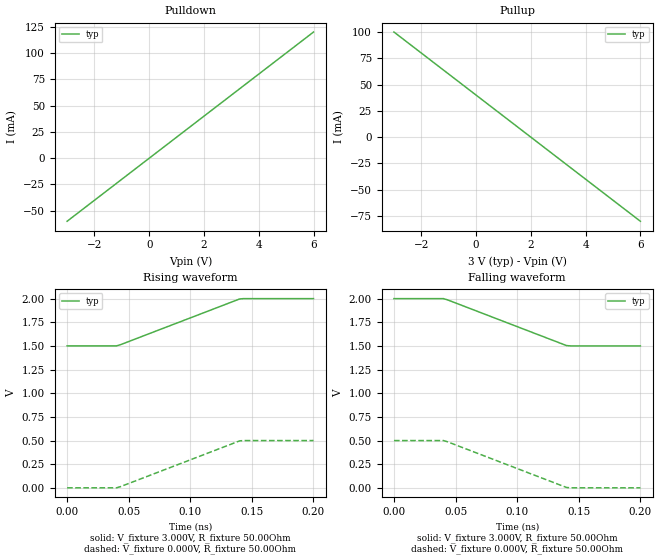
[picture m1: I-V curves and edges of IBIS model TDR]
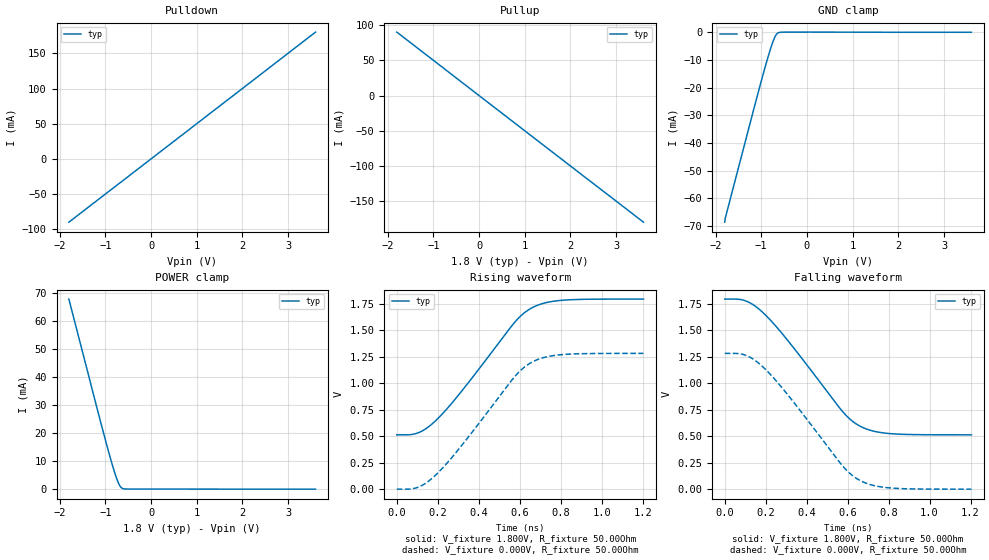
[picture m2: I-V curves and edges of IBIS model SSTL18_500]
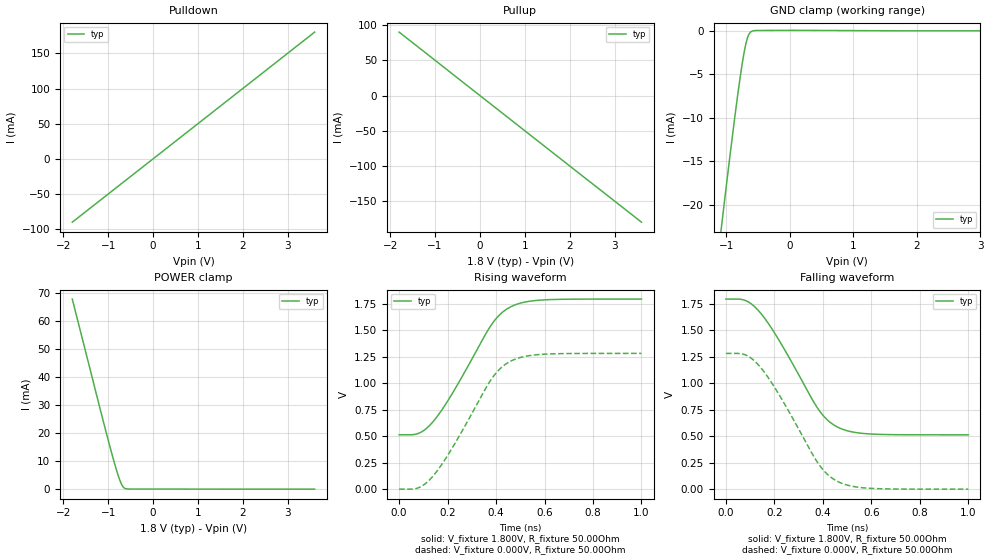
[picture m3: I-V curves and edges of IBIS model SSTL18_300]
[IBIS Ver]   3.2
[File Name]   bogatin_lab.ibs
[File Rev]   0.00
[Date]   10/29/2003
[Source]   Arpad Muranyi, Mentor Graphics
[Notes]   These models were made from the HyperLynx .MOD libraries
[Disclaimer]   This information is for educational purposes only.
[Copyright]   Copyright 2013, Mentor Graphics.  All Rights Reserved.
[Component]   Bogatin_Lab
[Manufacturer]  Mentor Graphics Corporation
[Package]
|   typ   min   max
R_pkg   0.00Ohm   0.00Ohm   0.00Ohm
L_pkg   0.00nH   0.00nH   0.00nH
C_pkg   0.00pF   0.00pF   0.00pF
[PIN]   signal_name   model_name   R_pin   L_pin   C_pin
1   Vcc   Power
2   GND   GND
3   TDR   TDR   10.000mOhm   2.000nH   0.800pF
4   SSTL18_500   SSTL18_500   10.000mOhm   0.050nH   0.050pF
5   SSTL18_300   SSTL18_300   10.000mOhm   0.050nH   0.050pF
6   SSTL18_200   SSTL18_200   10.000mOhm   0.050nH   0.050pF
7   CMOS33_UF8   CMOS33_UF8   10.000mOhm   0.050nH   0.050pF
8   CMOS33_UF_P   CMOS33_UF8   10.000mOhm   0.050nH   0.050pF
9   CMOS33_UF_N   CMOS33_UF8   10.000mOhm   0.050nH   0.050pF
10   CMOS33_UF4   CMOS33_UF4   10.000mOhm   2.000nH   0.800pF
11   CMOS33_UF4   CMOS33_UF4   10.000mOhm   0.050nH   0.050pF
12   CMOS33_MED8   CMOS33_MED8   10.000mOhm   0.050nH   0.050pF
13   CMOS33_MED4   CMOS33_MED4   10.000mOhm   0.050nH   0.050pF
14   SSTL25_01ns   SSTL25_01ns   10.000mOhm   0.050nH   0.050pF
[Diff Pin]  inv_pin  vdiff  tdelay_typ tdelay_min tdelay_max
 8   9   100mV   0ns   0ns   0ns
| Models and submodels in the file (9): TDR (Output), SSTL18_500 (I/O), SSTL18_300 (I/O), SSTL18_200 (I/O), CMOS33_UF8 (I/O), CMOS33_UF4 (I/O), CMOS33_MED8 (I/O), CMOS33_MED4 (I/O), SSTL25_01ns (I/O)
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[Model]   TDR
Model_type   Output
Vmeas = 1.500V
Vref = 0.000V
Cref = 50.000pF
Rref = 1.000kOhm
|   typ   min   max
C_comp   0.000F   NA   NA
[Voltage Range]   3.000V   NA   NA
[Temperature Range]   50.0   NA   NA
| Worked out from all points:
|   slope of the pulldown table from 0 to 0.45 V, typ, clamps not added: 50 ohm
|   slope of the pullup table from 0 to 0.45 V, typ, clamps not added: 50 ohm
|   falling waveform, V_fixture 3.000V, R_fixture 50.00Ohm: 20-80 % time 60ps typ, NA min, NA max; typ from 2 V to 1.5 V
|   rising waveform, V_fixture 3.000V, R_fixture 50.00Ohm: 20-80 % time 60ps typ, NA min, NA max; typ from 1.5 V to 2 V
|   rising waveform, V_fixture 0.000V, R_fixture 50.00Ohm: 20-80 % time 60ps typ, NA min, NA max; typ from 0 V to 0.5 V
|   falling waveform, V_fixture 0.000V, R_fixture 50.00Ohm: 20-80 % time 60ps typ, NA min, NA max; typ from 0.5 V to 0 V
[Pulldown]
|   Voltage   I(typ)   I(min)   I(max)
-3V       -60mA      NA         NA
6V        120mA      NA         NA
[Pullup]
|   Voltage   I(typ)   I(min)   I(max)
-3V       100mA      NA         NA
6V        -80mA      NA         NA
[Ramp]
R_load = 50.00Ohm
|   typ   min   max
dV/dt_r   300.000mV/60.000ps   NA   NA
dV/dt_f   300.000mV/60.000ps   NA   NA
[Falling Waveform]
V_fixture = 3.000V
R_fixture = 50.00Ohm
|   Time   V(typ)   V(min)   V(max)
0s        2V         NA         NA
40.08ps   2V         NA         NA
43.21ps   1.988V     NA         NA
46.34ps   1.973V     NA         NA
140.2ps   1.504V     NA         NA
143.5ps   1.5V       NA         NA
200ps     1.5V       NA         NA
[Rising Waveform]
V_fixture = 3.000V
R_fixture = 50.00Ohm
|   Time   V(typ)   V(min)   V(max)
0s        1.5V       NA         NA
40.08ps   1.5V       NA         NA
43.21ps   1.513V     NA         NA
46.34ps   1.528V     NA         NA
140.2ps   1.996V     NA         NA
143.5ps   2V         NA         NA
200ps     2V         NA         NA
[Rising Waveform]
V_fixture = 0.000V
R_fixture = 50.00Ohm
|   Time   V(typ)   V(min)   V(max)
0s        0V         NA         NA
40.08ps   98.81uV    NA         NA
43.21ps   12.23mV    NA         NA
46.34ps   27.67mV    NA         NA
140.2ps   496.4mV    NA         NA
143.5ps   499.8mV    NA         NA
200ps     500mV      NA         NA
[Falling Waveform]
V_fixture = 0.000V
R_fixture = 50.00Ohm
|   Time   V(typ)   V(min)   V(max)
0s        500mV      NA         NA
40.08ps   499.8mV    NA         NA
43.21ps   487.7mV    NA         NA
46.34ps   472.2mV    NA         NA
140.2ps   3.638mV    NA         NA
143.5ps   173.4uV    NA         NA
200ps     0V         NA         NA
[Model]   SSTL18_500
Model_type   I/O
Vinl = 650.000mV
Vinh = 1.150V
Vmeas = 900.000mV
Vref = 900.000mV
Cref = 100.000fF
Rref = 25.000Ohm
|   typ   min   max
C_comp   4.000pF   NA   NA
[Voltage Range]   1.800V   NA   NA
[Temperature Range]   50.0   NA   NA
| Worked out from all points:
|   slope of the pulldown table from 0 to 0.27 V, typ, clamps not added: 20 ohm
|   slope of the pullup table from 0 to 0.27 V, typ, clamps not added: 20 ohm
|   GND clamp passes 1 mA (typ) near -0.68 V on its own axis
|   POWER clamp passes 1 mA (typ) near -0.68 V on its own axis
|   falling waveform, V_fixture 1.800V, R_fixture 50.00Ohm: 20-80 % time 310ps typ, NA min, NA max; typ from 1.8 V to 0.512 V
|   rising waveform, V_fixture 1.800V, R_fixture 50.00Ohm: 20-80 % time 310ps typ, NA min, NA max; typ from 0.512 V to 1.8 V
|   rising waveform, V_fixture 0.000V, R_fixture 50.00Ohm: 20-80 % time 310ps typ, NA min, NA max; typ from -0.002 V to 1.28 V
|   falling waveform, V_fixture 0.000V, R_fixture 50.00Ohm: 20-80 % time 310ps typ, NA min, NA max; typ from 1.28 V to -0.002 V
[Pulldown]
|   Voltage   I(typ)   I(min)   I(max)
-1.8V     -89.85mA   NA         NA
-1.79V    -89.29mA   NA         NA
0V        83.28uA    NA         NA
3.6V      180.1mA    NA         NA
[GND Clamp]
|   Voltage   I(typ)   I(min)   I(max)
-1.8V     -68.65mA   NA         NA
-1.79V    -67.3mA    NA         NA
-1.17V    -28.2mA    NA         NA
-920mV    -12.89mA   NA         NA
-820mV    -7.212mA   NA         NA
-740mV    -3.24mA    NA         NA
-690mV    -1.365mA   NA         NA
-640mV    -324.9uA   NA         NA
-520mV    39.96uA    NA         NA
3.6V      0A         NA         NA
[Pullup]
|   Voltage   I(typ)   I(min)   I(max)
-1.8V     90.25mA    NA         NA
-810mV    40.79mA    NA         NA
1.8V      -89.88mA   NA         NA
3.6V      -179.7mA   NA         NA
[POWER Clamp]
|   Voltage   I(typ)   I(min)   I(max)
-1.8V     67.89mA    NA         NA
-1.12V    24.88mA    NA         NA
-900mV    11.56mA    NA         NA
-810mV    6.555mA    NA         NA
-750mV    3.62mA     NA         NA
-700mV    1.673mA    NA         NA
-650mV    514.2uA    NA         NA
-530mV    49.56uA    NA         NA
3.6V      0A         NA         NA
[Ramp]
R_load = 50.00Ohm
|   typ   min   max
dV/dt_r   771.100mV/310.137ps   NA   NA
dV/dt_f   771.043mV/310.137ps   NA   NA
[Falling Waveform]
V_fixture = 1.800V
R_fixture = 50.00Ohm
|   Time   V(typ)   V(min)   V(max)
0s        1.797V     NA         NA
101.7ps   1.781V     NA         NA
187.7ps   1.668V     NA         NA
308.9ps   1.403V     NA         NA
574.8ps   734.3mV    NA         NA
615.9ps   653.6mV    NA         NA
656.9ps   598.3mV    NA         NA
723.4ps   548.8mV    NA         NA
809.4ps   523.6mV    NA         NA
1.204ns   512.3mV    NA         NA
[Rising Waveform]
V_fixture = 1.800V
R_fixture = 50.00Ohm
|   Time   V(typ)   V(min)   V(max)
0s        512.3mV    NA         NA
101.7ps   529.4mV    NA         NA
187.7ps   642.4mV    NA         NA
308.9ps   907mV      NA         NA
574.8ps   1.575V     NA         NA
615.9ps   1.656V     NA         NA
656.9ps   1.711V     NA         NA
723.4ps   1.761V     NA         NA
809.4ps   1.786V     NA         NA
1.204ns   1.797V     NA         NA
[Rising Waveform]
V_fixture = 0.000V
R_fixture = 50.00Ohm
|   Time   V(typ)   V(min)   V(max)
0s        -2.064mV   NA         NA
101.7ps   14.81mV    NA         NA
187.7ps   127.8mV    NA         NA
308.9ps   392.4mV    NA         NA
574.8ps   1.061V     NA         NA
615.9ps   1.142V     NA         NA
656.9ps   1.197V     NA         NA
723.4ps   1.247V     NA         NA
809.4ps   1.272V     NA         NA
1.204ns   1.283V     NA         NA
[Falling Waveform]
V_fixture = 0.000V
R_fixture = 50.00Ohm
|   Time   V(typ)   V(min)   V(max)
0s        1.283V     NA         NA
101.7ps   1.266V     NA         NA
187.7ps   1.153V     NA         NA
308.9ps   888.4mV    NA         NA
574.8ps   219.9mV    NA         NA
615.9ps   139.2mV    NA         NA
656.9ps   83.94mV    NA         NA
723.4ps   34.39mV    NA         NA
809.4ps   9.174mV    NA         NA
1.204ns   -2.064mV   NA         NA
[Model]   SSTL18_300
Model_type   I/O
Vinl = 650.000mV
Vinh = 1.150V
Vmeas = 900.000mV
Vref = 900.000mV
Cref = 100.000fF
Rref = 25.000Ohm
|   typ   min   max
C_comp   4.000pF   NA   NA
[Voltage Range]   1.800V   NA   NA
[Temperature Range]   50.0   NA   NA
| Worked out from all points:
|   slope of the pulldown table from 0 to 0.27 V, typ, clamps not added: 20 ohm
|   slope of the pullup table from 0 to 0.27 V, typ, clamps not added: 20 ohm
|   GND clamp passes 1 mA (typ) near -0.68 V on its own axis
|   POWER clamp passes 1 mA (typ) near -0.68 V on its own axis
|   falling waveform, V_fixture 1.800V, R_fixture 50.00Ohm: 20-80 % time 194ps typ, NA min, NA max; typ from 1.8 V to 0.512 V
|   rising waveform, V_fixture 1.800V, R_fixture 50.00Ohm: 20-80 % time 194ps typ, NA min, NA max; typ from 0.512 V to 1.8 V
|   rising waveform, V_fixture 0.000V, R_fixture 50.00Ohm: 20-80 % time 194ps typ, NA min, NA max; typ from -0.002 V to 1.28 V
|   falling waveform, V_fixture 0.000V, R_fixture 50.00Ohm: 20-80 % time 194ps typ, NA min, NA max; typ from 1.28 V to -0.002 V
[Pulldown]
|   Voltage   I(typ)   I(min)   I(max)
-1.8V     -89.85mA   NA         NA
-1.79V    -89.29mA   NA         NA
0V        83.31uA    NA         NA
3.6V      180.1mA    NA         NA
[GND Clamp]
|   Voltage   I(typ)   I(min)   I(max)
-1.8V     -68.65mA   NA         NA
-1.09V    -23.21mA   NA         NA
-1.07V    -21.97mA   NA         NA
-880mV    -10.56mA   NA         NA
-820mV    -7.212mA   NA         NA
-760mV    -4.154mA   NA         NA
-720mV    -2.411mA   NA         NA
-680mV    -1.082mA   NA         NA
-650mV    -459.3uA   NA         NA
-610mV    -90.03uA   NA         NA
0V        59.41uA    NA         NA
3.6V      0A         NA         NA
[Pullup]
|   Voltage   I(typ)   I(min)   I(max)
-1.8V     90.25mA    NA         NA
-810mV    40.79mA    NA         NA
1.8V      -89.88mA   NA         NA
3.6V      -179.7mA   NA         NA
[POWER Clamp]
|   Voltage   I(typ)   I(min)   I(max)
-1.8V     67.89mA    NA         NA
-1.12V    24.88mA    NA         NA
-900mV    11.56mA    NA         NA
-810mV    6.555mA    NA         NA
-750mV    3.62mA     NA         NA
-700mV    1.673mA    NA         NA
-650mV    514.2uA    NA         NA
-530mV    49.61uA    NA         NA
3.6V      0A         NA         NA
[Ramp]
R_load = 50.00Ohm
|   typ   min   max
dV/dt_r   771.100mV/194.169ps   NA   NA
dV/dt_f   771.043mV/194.169ps   NA   NA
[Falling Waveform]
V_fixture = 1.800V
R_fixture = 50.00Ohm
|   Time   V(typ)   V(min)   V(max)
0s        1.797V     NA         NA
79.18ps   1.785V     NA         NA
138.8ps   1.676V     NA         NA
218ps     1.412V     NA         NA
377.3ps   767.9mV    NA         NA
413.5ps   664.6mV    NA         NA
453.6ps   594.2mV    NA         NA
510.3ps   545.2mV    NA         NA
588.5ps   521.4mV    NA         NA
1ns       512.3mV    NA         NA
[Rising Waveform]
V_fixture = 1.800V
R_fixture = 50.00Ohm
|   Time   V(typ)   V(min)   V(max)
0s        512.3mV    NA         NA
79.18ps   525.4mV    NA         NA
138.8ps   633.5mV    NA         NA
218ps     897.9mV    NA         NA
377.3ps   1.542V     NA         NA
413.5ps   1.645V     NA         NA
453.6ps   1.715V     NA         NA
510.3ps   1.764V     NA         NA
589.5ps   1.788V     NA         NA
1ns       1.797V     NA         NA
[Rising Waveform]
V_fixture = 0.000V
R_fixture = 50.00Ohm
|   Time   V(typ)   V(min)   V(max)
0s        -2.064mV   NA         NA
79.18ps   10.77mV    NA         NA
138.8ps   118.9mV    NA         NA
218ps     383.3mV    NA         NA
377.3ps   1.027V     NA         NA
413.5ps   1.131V     NA         NA
453.6ps   1.201V     NA         NA
509.3ps   1.25V      NA         NA
588.5ps   1.274V     NA         NA
1ns       1.283V     NA         NA
[Falling Waveform]
V_fixture = 0.000V
R_fixture = 50.00Ohm
|   Time   V(typ)   V(min)   V(max)
0s        1.283V     NA         NA
79.18ps   1.27V      NA         NA
138.8ps   1.162V     NA         NA
218ps     897.5mV    NA         NA
377.3ps   253.5mV    NA         NA
413.5ps   150.2mV    NA         NA
453.6ps   79.84mV    NA         NA
510.3ps   30.85mV    NA         NA
588.5ps   6.977mV    NA         NA
1ns       -2.064mV   NA         NA
